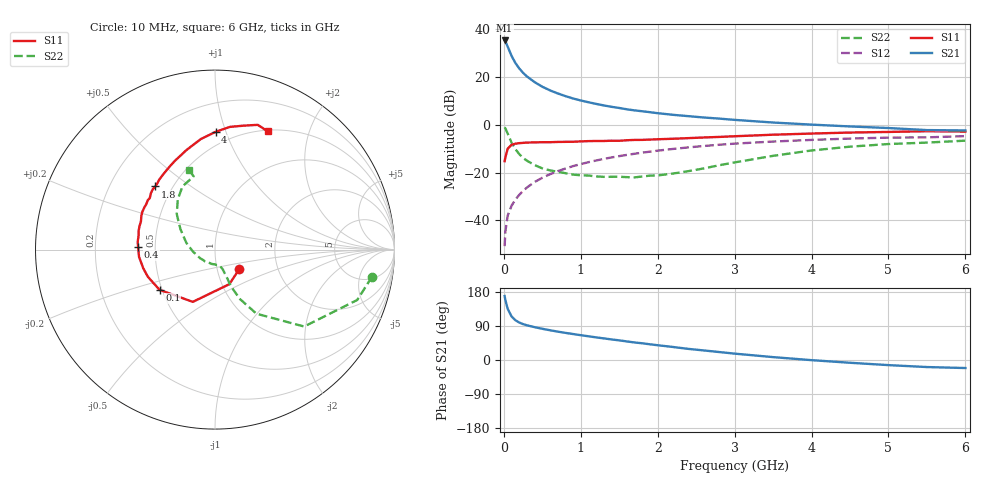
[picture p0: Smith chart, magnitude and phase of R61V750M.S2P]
! SIEMENS Small Signal Semiconductors
! BFR193
! Si NPN RF Bipolar Junction Transistor in SOT23
! VCE = 1.75 V  IC = 50 mA
! Common Emitter S-Parameters:  May  1996
# GHz  S  MA  R  50
!  f  S11  S21  S12  S22
! GHz  MAG  ANG  MAG  ANG  MAG  ANG  MAG  ANG
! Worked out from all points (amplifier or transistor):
!   36 points, 10 MHz to 6 GHz, reference 50 ohm
!   highest |S21| = 35.3 dB at 10 MHz (marker M1)
!   |S21| within 3 dB of that: start of sweep to 55.56 MHz
!   unconditionally stable (mu >= 1): 337.6 MHz to 2.022 GHz
!   at 250 MHz: K = 0.97, MSG = 24.7 dB, |S12| = -27.6 dB
!   at 1.4 GHz: K = 1.02, MAG = 9.6 dB, |S12| = -13.7 dB
!   at 6 GHz: K = 0.96, MSG = 1.2 dB, |S12| = -4.7 dB
!   S11 on the Smith chart (normalised r, x): 10 MHz: 1.28, -0.28; 100 MHz: 0.48, -0.25; 400 MHz: 0.40, +0.01; 1.8 GHz: 0.40, +0.37; 4 GHz: 0.40, +0.92; 6 GHz: 0.51, +1.41
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0.01  0.1734 -38.3  58.02 168.8  0.0029 83.8  0.8879 -9.8
0.02  0.2086 -67.5  55.46 158.3  0.0059 78.7  0.8407 -19.5
0.05  0.3164 -113.0  43.15 134.9  0.0126 68.4  0.6559 -40.8
0.1  0.3815 -144.0  27.68 115.1  0.0203 68.9  0.4254 -57.1
0.15  0.4034 -157.9  19.62 104.9  0.0273 70.1  0.3102 -63.1
0.2  0.4131 -165.4  15.11 98.9  0.0343 72.1  0.2447 -65.5
0.25  0.4193 -171.2  12.22 94.7  0.0415 73.4  0.2032 -66.8
0.3  0.4252 -174.6  10.26 91.6  0.0488 74.2  0.1778 -66.8
0.4  0.4288 178.1  7.798 86.7  0.0637 74.5  0.1438 -67.7
0.5  0.4329 174.2  6.255 82.4  0.078 74.2  0.1227 -68.4
0.6  0.4327 169.7  5.25 78.5  0.0927 73.3  0.1114 -69.3
0.7  0.4382 166.1  4.533 74.9  0.1072 72.5  0.1043 -71.1
0.9  0.4419 158.9  3.549 68.5  0.1368 69.9  0.0909 -75.9
1.1  0.456 152.9  2.96 62.6  0.1653 67.2  0.0869 -83.9
1.4  0.4647 143.7  2.376 54.3  0.2076 62.8  0.0818 -97.4
1.8  0.4839 133.3  1.919 44.1  0.2617 56.5  0.0831 -121.6
2.2  0.5111 123.8  1.617 34.3  0.313 50.2  0.0958 -149.7
3.5  0.621 97.3  1.116 7.6  0.4465 29.0  0.2245 149.2
4  0.6561 89.7  1.009 -0.4  0.4832 21.8  0.2909 137.1
4.5  0.6886 83.1  0.924 -7.3  0.5156 14.7  0.3491 126.4
5.5  0.7347 71.1  0.775 -18.6  0.5465 1.0  0.4248 106.3
6  0.7217 66.0  0.763 -21.2  0.5801 -3.0  0.4663 107.9
